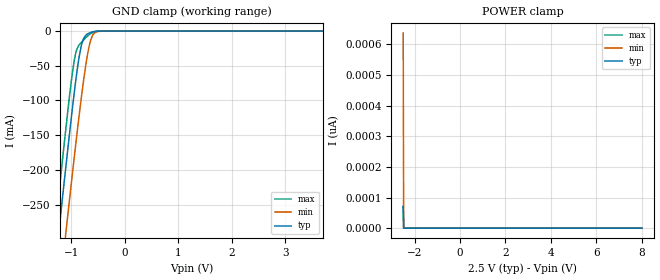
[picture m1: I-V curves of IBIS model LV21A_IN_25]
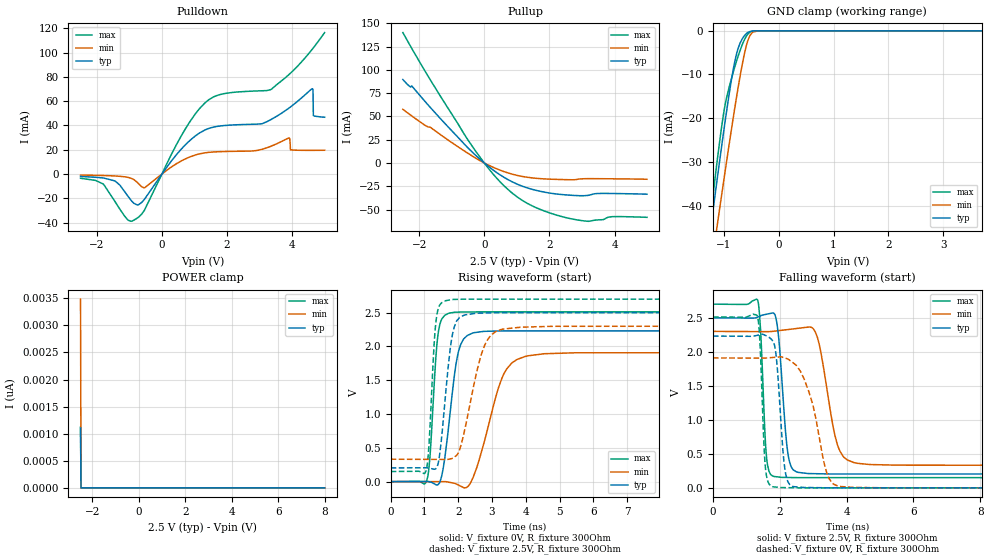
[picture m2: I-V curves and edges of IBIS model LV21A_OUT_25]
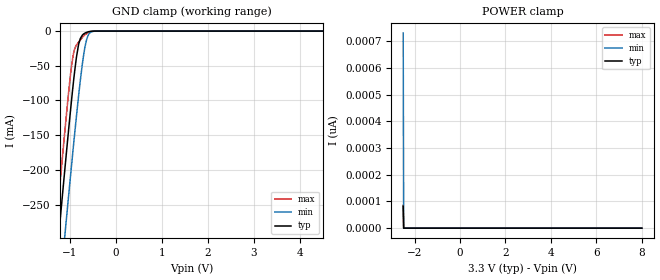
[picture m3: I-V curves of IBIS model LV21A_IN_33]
| TEXAS INSTRUMENTS INCORPORATED
| Standard Linear and Logic Group
| IBIS Model of SN74LV21A
[IBIS Ver]   3.2
[Comment Char]  |_char
[File Name]   lv21a.ibs
[File Rev]   2.0 I_die
[Date]   Febraury 25, 2022
[Source]   Data created from HSPICE simulations at TI-SLL.
[Notes]   The following is an IBIS list for the LV21A.
|   Please contact sllibis@ti.com with questions and
|   comments concerning SLL IBIS models.
|   The warning about AC Rising Endpoint might be reported,
|   but it is due to HSPICE issue and negligible.
[Disclaimer] Property of Texas Instruments Incorporated.  Unauthorized
   reproduction and/or distribution is strictly prohibited.
   This product is protected under copyright law.
   Created 2022, (C) Copyright 2022, Texas Instruments Inc.,
   All Rights Reserved.
   UNLESS THERE IS A SIGNED, WRITTEN AGREEMENT TO THE
   CONTRARY, TEXAS INSTRUMENTS () IS PROVIDING THE IBIS
   MODELS  AND WITHOUT ANY WARRANTY, EXPRESSED OR
   IMPLIED.  TI assumes no liability for:
   1) the accuracy of the IBIS models provided to your
   company;
   2) the proper functioning of these IBIS Models in your
   design or for any resulting applications; or
   3) infringement of patents, copyrights or intellectual
   property rights resulting from your use of these IBIS
   models.
   TI provides IBIS Models as a service to our customers.
   You and your company shall not distribute, sell or give
   these models to anyone else without prior written
   permission from TI.
   TI reserves the right to make changes to our products or
   to discontinue any semiconductor product or service
   without notice, and advises our customers to obtain the
   latest version of relevant information to verify, before
   placing orders, that the information being relied on is
   current.
   Please be aware that your receipt and use of the IBIS
   information provided shall serve as acceptance of these
   terms and conditions.  If you do not accept these terms,
   you should return or destroy the IBIS models and any
   other accompanying information immediately.
|   Component LV21A_D
[Component]   LV21A_D
[Manufacturer]  Texas Instruments, Inc.
[Package]
|   typ   min   max
R_pkg   0.031   0.028   0.034
L_pkg   3.109nH   2.462nH   3.889nH
C_pkg   0.473pF   0.363pF   0.628pF
[Pin]   signal_name   model_name   R_pin   L_pin   C_pin
1   1A   LV21A_IN   0.033   3.854nH   0.622pF
2   1B   LV21A_IN   0.032   3.188nH   0.473pF
3   1Y   LV21A_OUT   0.028   2.462nH   0.377pF
4   2A   LV21A_IN   0.031   2.596nH   0.363pF
5   2B   LV21A_IN   0.028   2.521nH   0.372pF
6   2Y   LV21A_OUT   0.034   3.250nH   0.476pF
7   GND   GND   0.034   3.889nH   0.628pF
8   3Y   LV21A_OUT   0.034   3.889nH   0.628pF
9   3A   LV21A_IN   0.034   3.250nH   0.476pF
10   3B   LV21A_IN   0.028   2.521nH   0.372pF
11   4Y   LV21A_OUT   0.031   2.596nH   0.364pF
12   4A   LV21A_IN   0.028   2.462nH   0.377pF
13   4B   LV21A_IN   0.032   3.188nH   0.473pF
14   VCC   POWER   0.033   3.854nH   0.622pF
|   Component LV21A_PW
[Component]   LV21A_PW
[Manufacturer]  Texas Instruments, Inc.
[Package]
|   typ   min   max
R_pkg   0.032   0.029   0.035
L_pkg   2.378nH   2.170nH   2.680nH
C_pkg   0.314pF   0.270pF   0.335pF
[Pin]   signal_name   model_name   R_pin   L_pin   C_pin
1   1A   LV21A_IN   0.033   2.618nH   0.330pF
2   1B   LV21A_IN   0.031   2.313nH   0.317pF
3   1Y   LV21A_OUT   0.030   2.310nH   0.314pF
4   2A   LV21A_IN   0.031   2.173nH   0.272pF
5   2B   LV21A_IN   0.030   2.204nH   0.309pF
6   2Y   LV21A_OUT   0.032   2.315nH   0.317pF
7   GND   GND   0.035   2.680nH   0.335pF
8   3Y   LV21A_OUT   0.033   2.640nH   0.333pF
9   3A   LV21A_IN   0.034   2.347nH   0.319pF
10   3B   LV21A_IN   0.029   2.277nH   0.313pF
11   4Y   LV21A_OUT   0.031   2.170nH   0.270pF
12   4A   LV21A_IN   0.031   2.244nH   0.311pF
13   4B   LV21A_IN   0.033   2.343nH   0.321pF
14   VCC   POWER   0.035   2.657nH   0.332pF
[Model Selector]   LV21A_IN
LV21A_IN_25   2.5-V Vcc Input Model
LV21A_IN_33   3.3-V Vcc Input Model
LV21A_IN_50   5.0-V Vcc Input Model
[Model Selector]   LV21A_OUT
LV21A_OUT_25   2.5-V Vcc Output Model
LV21A_OUT_33   3.3-V Vcc Output Model
LV21A_OUT_50   5.0-V Vcc Output Model
| Models and submodels in the file (6): LV21A_IN_25 (Input), LV21A_OUT_25 (Output), LV21A_IN_33 (Input), LV21A_OUT_33 (Output), LV21A_IN_50 (Input), LV21A_OUT_50 (Output)
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|   Model LV21A_IN_25
[Model]   LV21A_IN_25
Model_type   Input
Vinl = 0.75
Vinh = 1.75
|   typ   min   max
C_comp   3.5pF   3.4pF   3.7pF
[Voltage Range]   2.5   2.3   2.7
[Temperature Range]   25   125   -40
[Power Clamp Reference]   2.5   2.3   2.7
[GND Clamp Reference]   0   0   0
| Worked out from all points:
|   GND clamp passes 1 mA (typ) near -0.59 V on its own axis
[GND Clamp]
|   Voltage   I(typ)   I(min)   I(max)
-2.5V     -1.244A    -1.327A    -1.203A
-1.313V   -350.3mA   -444.6mA   -296.5mA
-1.23V    -289mA     -383.9mA   -234.5mA
-1.125V   -213.4mA   -308.8mA   -158.5mA
-1.072V   -176.4mA   -271.7mA   -121.6mA
-977.5mV  -111.7mA   -206mA     -60.6mA
-914.5mV  -71.44mA   -163.3mA   -31.85mA
-799mV    -17.49mA   -89.06mA   -15.38mA
-704.5mV  -4.594mA   -38.07mA   -7.858mA
-631mV    -1.797mA   -12.21mA   -3.542mA
-442mV    -17.94uA   -111.5uA   -18.13uA
8V        0A         0A         0A
[POWER Clamp]
|   Voltage   I(typ)   I(min)   I(max)
-2.5V     69.79pA    637.9pA    71.28pA
-2.479V   0A         0A         0A
-1mV      0A         0A         0A
8V        0A         0A         0A
|   Model LV21A_OUT_25
[Model]   LV21A_OUT_25
Model_type   Output
Polarity   Non-Inverting
Vmeas = 1.25
Vref = 0
Cref = 2pF
Rref = 100000
|   typ   min   max
C_comp   5.7pF   5.6pF   6pF
[Voltage Range]   2.5   2.3   2.7
[Temperature Range]   25   125   -40
[Pullup Reference]   2.5   2.3   2.7
[Pulldown Reference]   0   0   0
[Power Clamp Reference]   2.5   2.3   2.7
[GND Clamp Reference]   0   0   0
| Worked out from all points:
|   slope of the pulldown table from 0 to 0.375 V, typ, clamps not added: 27.6 ohm
|   slope of the pullup table from 0 to 0.375 V, typ, clamps not added: 37 ohm
|   GND clamp passes 1 mA (typ) near -0.62 V on its own axis
|   falling waveform, V_fixture 2.5V, R_fixture 300Ohm: 20-80 % time 207ps typ, 415ps min, 133ps max; typ from 2.5 V to 0.203 V
|   rising waveform, V_fixture 0V, R_fixture 300Ohm: 20-80 % time 324ps typ, 637ps min, 184ps max; typ from 0 V to 2.23 V
|   rising waveform, V_fixture 2.5V, R_fixture 300Ohm: 20-80 % time 274ps typ, 527ps min, 161ps max; typ from 0.203 V to 2.5 V
|   falling waveform, V_fixture 0V, R_fixture 300Ohm: 20-80 % time 191ps typ, 536ps min, 122ps max; typ from 2.23 V to 0 V
[Pulldown]
|   Voltage   I(typ)   I(min)   I(max)
-2.5V     -1.981mA   -826.2uA   -3.454mA
-1.45V    -5.598mA   -1.547mA   -22.23mA
-862mV    -24.03mA   -4.577mA   -37.93mA
-536.5mV  -20.75mA   -11.35mA   -29.7mA
1.312V    36.14mA    17.43mA    58.29mA
3.338V    44.71mA    22.77mA    69.46mA
3.905V    54.39mA    29.66mA    81.96mA
3.947V    55.23mA    19.9mA     83mA
4.619V    70.24mA    19.53mA    102.8mA
4.64V     69.48mA    19.53mA    103.5mA
4.651V    48.14mA    19.53mA    103.9mA
4.997V    46.76mA    19.6mA     116.4mA
[GND Clamp]
|   Voltage   I(typ)   I(min)   I(max)
-2.5V     -170.7mA   -168.9mA   -187.4mA
-1.282V   -49.09mA   -58.54mA   -46.61mA
-1.24V    -45.04mA   -54.83mA   -42.02mA
-1.208V   -42.02mA   -52.06mA   -38.61mA
-1.125V   -34.05mA   -44.71mA   -29.82mA
-977.5mV  -20.62mA   -32.07mA   -16.86mA
-799mV    -6.847mA   -17.4mA    -8.124mA
-715mV    -3.091mA   -11.05mA   -4.817mA
-641.5mV  -1.357mA   -6.134mA   -2.454mA
-526mV    -161.3uA   -1.092mA   -287.1uA
-379mV    -1.458uA   -24.14uA   -787.4nA
8V        0A         0A         0A
[Pullup]
|   Voltage   I(typ)   I(min)   I(max)
-2.5V     89.57mA    57.59mA    140mA
-2.269V   81.68mA    51.57mA    125.6mA
-2.216V   82.27mA    50.23mA    122.4mA
-1.335V   47.15mA    30.14mA    70.99mA
-253mV    7.827mA    4.954mA    12.12mA
429.5mV   -11.45mA   -6.948mA   -18.12mA
1.018V    -22.83mA   -13.4mA    -36.6mA
1.899V    -31.65mA   -17.2mA    -52.27mA
2.929V    -35.16mA   -17.19mA   -61.54mA
3.223V    -34.57mA   -16.84mA   -62.58mA
3.958V    -32.78mA   -17.01mA   -57.61mA
4.997V    -33.52mA   -17.49mA   -58.36mA
[POWER Clamp]
|   Voltage   I(typ)   I(min)   I(max)
-2.5V     1.103nA    3.484nA    1.124nA
-2.479V   0A         0A         0A
-2.469V   0A         0A         0A
8V        0A         0A         0A
[Ramp]
R_load = 300
|   typ   min   max
dV/dt_r   1.33848/3.2081e-10   1.14527/6.3474e-10   1.50716/1.83481e-10
dV/dt_f   1.37803/2.06682e-10   1.18099/4.12383e-10   1.53027/1.33173e-10
[Falling Waveform]
V_fixture = 2.5V
V_fixture_min = 2.3V
V_fixture_max = 2.7V
R_fixture = 300Ohm
C_fixture = 0F
|   Time   V(typ)   V(min)   V(max)
0s        2.5V       2.3V       2.7V
1.336ns   2.51V      2.297V     2.762V
1.597ns   2.552V     2.296V     479.9mV
1.794ns   2.571V     2.3V       171.7mV
2.237ns   524mV      2.327V     152.7mV
2.501ns   234.6mV    2.342V     150.5mV
3.062ns   208.3mV    2.292V     149.9mV
3.714ns   204mV      651.4mV    149.9mV
4.219ns   204mV      371.3mV    149.9mV
15ns      203.3mV    331.7mV    149.5mV
[Rising Waveform]
V_fixture = 0V
V_fixture_min = 0V
V_fixture_max = 0V
R_fixture = 300Ohm
C_fixture = 0F
|   Time   V(typ)   V(min)   V(max)
0s        3.685uV    391.8nV    5.336uV
1.068ns   3.232mV    -66.86uV   16.97mV
1.165ns   -4.721mV   -96.64uV   376.2mV
1.403ns   -44.26mV   -169.7uV   2.177V
1.71ns    788.6mV    -7.387mV   2.489V
1.937ns   1.746V     -33.2mV    2.507V
2.163ns   2.111V     -88.82mV   2.51V
3.333ns   2.229V     1.575V     2.511V
3.975ns   2.229V     1.851V     2.511V
15ns      2.231V     1.909V     2.512V
[Rising Waveform]
V_fixture = 2.5V
V_fixture_min = 2.3V
V_fixture_max = 2.7V
R_fixture = 300Ohm
C_fixture = 0F
|   Time   V(typ)   V(min)   V(max)
0s        203.3mV    331.7mV    149.5mV
1.046ns   205.2mV    329.5mV    159mV
1.133ns   199.2mV    329.3mV    533.6mV
1.343ns   195.3mV    328.8mV    2.375V
1.622ns   1.267V     328.2mV    2.675V
1.791ns   2.063V     339.5mV    2.692V
1.962ns   2.383V     394.1mV    2.697V
2.736ns   2.494V     1.957V     2.7V
3.273ns   2.499V     2.251V     2.7V
15ns      2.5V       2.3V       2.7V
[Falling Waveform]
|Gnd
V_fixture = 0V
V_fixture_min = 0V
V_fixture_max = 0V
R_fixture = 300Ohm
C_fixture = 0F
|   Time   V(typ)   V(min)   V(max)
0s        2.231V     1.909V     2.512V
1.329ns   2.242V     1.908V     2.525V
1.403ns   2.25V      1.908V     2.16V
1.557ns   2.243V     1.907V     364.7mV
1.753ns   2.181V     1.915V     20.31mV
1.894ns   1.928V     1.92V      10.93mV
2.149ns   284.5mV    1.909V     3.535mV
2.375ns   23.02mV    1.846V     1.807mV
3.745ns   611.5uV    25.96mV    289.8uV
15ns      4.24uV     1.273uV    5.484uV
|   Model LV21A_IN_33
[Model]   LV21A_IN_33
Model_type   Input
Vinl = 0.99
Vinh = 2.31
|   typ   min   max
C_comp   3.5pF   3.4pF   3.7pF
[Voltage Range]   3.3   3   3.6
[Temperature Range]   25   125   -40
[Power Clamp Reference]   3.3   3   3.6
[GND Clamp Reference]   0   0   0
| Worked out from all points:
|   GND clamp passes 1 mA (typ) near -0.59 V on its own axis
[GND Clamp]
|   Voltage   I(typ)   I(min)   I(max)
-2.5V     -1.244A    -1.327A    -1.203A
-1.313V   -350.3mA   -444.6mA   -296.5mA
-1.23V    -289mA     -383.9mA   -234.5mA
-1.125V   -213.4mA   -308.8mA   -158.5mA
-1.072V   -176.4mA   -271.7mA   -121.6mA
-977.5mV  -111.7mA   -206mA     -60.6mA
-914.5mV  -71.44mA   -163.3mA   -31.85mA
-799mV    -17.49mA   -89.06mA   -15.38mA
-704.5mV  -4.594mA   -38.07mA   -7.858mA
-631mV    -1.797mA   -12.21mA   -3.542mA
-442mV    -17.94uA   -111.5uA   -18.13uA
8V        0A         0A         0A
[POWER Clamp]
|   Voltage   I(typ)   I(min)   I(max)
-2.5V     82.14pA    731.9pA    85.63pA
-2.479V   0A         0A         0A
-1mV      0A         0A         0A
8V        0A         0A         0A
